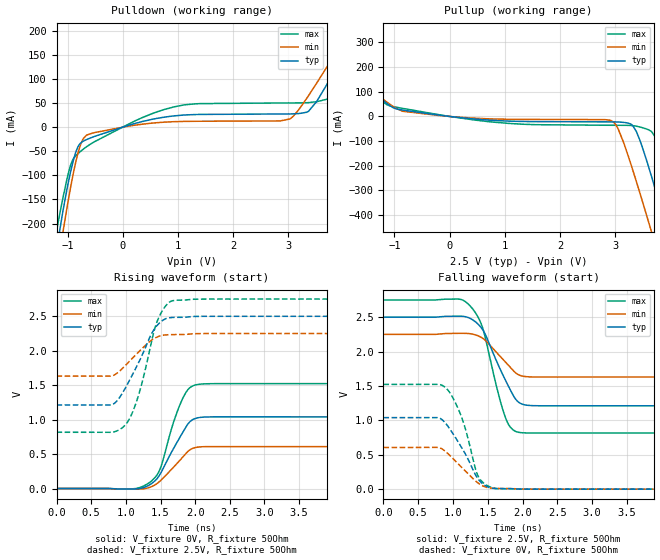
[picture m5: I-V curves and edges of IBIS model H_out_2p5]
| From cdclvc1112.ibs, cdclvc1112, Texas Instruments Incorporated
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|   H_out_2p5
[Model]   H_out_2p5
|Signals :   Y0, Y1, Y2, Y3, Y4, Y5, Y6, Y7, Y8 and Y9
Model_type   Output
Polarity   Non-Inverting
Enable   Active-Low
Vmeas   = 1.21
Vref   = 1.25
Cref   = 2pF
Rref   = 50
|   typ   min   max
C_comp   283fF   269fF   303fF
|C_comp (High state)   176fF   174fF   179fF
[Voltage Range]   2.5   2.25   2.75
[Temperature Range]   25   85   -40
[Pullup Reference]   2.5   2.25   2.75
[Pulldown Reference]   0   0   0
[Power Clamp Reference]   2.5   2.25   2.75
[GND Clamp Reference]   0   0   0
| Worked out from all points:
|   slope of the pulldown table from 0 to 0.375 V, typ, clamps not added: 30.7 ohm
|   slope of the pullup table from 0 to 0.375 V, typ, clamps not added: 43.2 ohm
|   falling waveform, V_fixture 2.5V, R_fixture 50Ohm: 20-80 % time 342ps typ, 337ps min, 282ps max; typ from 2.5 V to 1.21 V
|   rising waveform, V_fixture 0V, R_fixture 50Ohm: 20-80 % time 336ps typ, 340ps min, 279ps max; typ from 0 V to 1.04 V
|   rising waveform, V_fixture 2.5V, R_fixture 50Ohm: 20-80 % time 369ps typ, 373ps min, 297ps max; typ from 1.21 V to 2.5 V
|   falling waveform, V_fixture 0V, R_fixture 50Ohm: 20-80 % time 341ps typ, 361ps min, 268ps max; typ from 1.04 V to 0 V
[Pulldown]
|   Voltage   I(typ)   I(min)   I(max)
-2.5V     -1.296A    -1.308A    -1.284A
-1.206V   -260.7mA   -305.4mA   -220mA
-1.083V   -173.1mA   -216.7mA   -146mA
-853.8mV  -52.8mA    -73.62mA   -59.56mA
-655mV    -25.65mA   -16.52mA   -40.48mA
935mV     23.4mA     11.34mA    42.16mA
3.031V    27.38mA    16.98mA    50.17mA
3.369V    32.99mA    65.5mA     50.86mA
3.71V     90.55mA    126.6mA    58.62mA
4.149V    181.8mA    208.1mA    149.2mA
4.468V    250.2mA    268.2mA    226.3mA
5V        366.5mA    369.8mA    359.1mA
[Pullup]
|   Voltage   I(typ)   I(min)   I(max)
-2.5V     335.9mA    308.3mA    362.8mA
-1.094V   45.6mA     51.2mA     43.52mA
-846.2mV  25.65mA    20.9mA     32.57mA
42.5mV    -1.118mA   -792.6uA   -1.507mA
2.919V    -22.05mA   -15.77mA   -35.77mA
3.065V    -22.61mA   -55.91mA   -35.87mA
3.324V    -38.7mA    -220.3mA   -37.41mA
3.601V    -200.6mA   -424.3mA   -53.6mA
3.732V    -298.6mA   -523.9mA   -87.55mA
3.954V    -470.4mA   -694.2mA   -239.8mA
4.242V    -700.7mA   -919.5mA   -471.5mA
5V        -1.319A    -1.52A     -1.108A
[Ramp]
R_load = 50
|   typ   min   max
dV/dt_r   0.623775/3.36203e-010  0.363855/3.39637e-010  0.913559/2.7929e-010
dV/dt_f   0.772486/3.42455e-010  0.371071/3.371e-010   1.16011/2.82136e-010
[Falling Waveform]
V_fixture = 2.5V
V_fixture_min = 2.25V
V_fixture_max = 2.75V
R_fixture = 50Ohm
C_fixture = 0F
|   Time   V(typ)   V(min)   V(max)
0s        2.5V       2.25V      2.75V
1.072ns   2.514V     2.265V     2.763V
1.23ns    2.49V      2.261V     2.68V
1.425ns   2.32V      2.194V     2.347V
1.643ns   1.824V     1.969V     1.425V
1.755ns   1.581V     1.846V     1.037V
1.823ns   1.445V     1.772V     904.4mV
1.92ns    1.285V     1.676V     832.1mV
2.243ns   1.212V     1.63V      816.4mV
6.248ns   1.213V     1.632V     816.5mV
[Rising Waveform]
V_fixture = 0V
V_fixture_min = 0V
V_fixture_max = 0V
R_fixture = 50Ohm
C_fixture = 0F
|   Time   V(typ)   V(min)   V(max)
0s        3.877nV    3.665nV    2.043nV
1.103ns   -7.291mV   -9.573mV   -3.896mV
1.35ns    57.44mV    18.83mV    93.48mV
1.432ns   123.9mV    60.05mV    174.1mV
1.5ns     217.5mV    114.5mV    299.2mV
1.68ns    565.9mV    300.6mV    936.4mV
1.815ns   804.7mV    449.3mV    1.296V
1.905ns   948.5mV    546.4mV    1.445V
2.01ns    1.019V     595.8mV    1.505V
6.248ns   1.04V      606.4mV    1.523V
[Rising Waveform]
V_fixture = 2.5V
V_fixture_min = 2.25V
V_fixture_max = 2.75V
R_fixture = 50Ohm
C_fixture = 0F
|   Time   V(typ)   V(min)   V(max)
0s        1.213V     1.632V     816.5mV
795ps     1.216V     1.634V     816.3mV
990ps     1.453V     1.783V     920.5mV
1.08ns    1.623V     1.876V     1.069V
1.177ns   1.815V     1.975V     1.336V
1.357ns   2.221V     2.144V     2.072V
1.448ns   2.362V     2.197V     2.414V
1.552ns   2.454V     2.227V     2.621V
1.665ns   2.482V     2.234V     2.723V
6.248ns   2.5V       2.25V      2.75V
[Falling Waveform]
|Gnd
V_fixture = 0V
V_fixture_min = 0V
V_fixture_max = 0V
R_fixture = 50Ohm
C_fixture = 0F
|   Time   V(typ)   V(min)   V(max)
0s        1.04V      606.4mV    1.523V
772.5ps   1.04V      606.5mV    1.524V
900ps     949.7mV    541.5mV    1.468V
1.012ns   786mV      431.6mV    1.301V
1.125ns   603.1mV    316.5mV    1.042V
1.32ns    215.1mV    122.4mV    305.6mV
1.357ns   152.9mV    91.38mV    199.3mV
1.448ns   62.24mV    38.73mV    82.87mV
1.583ns   12.29mV    12.39mV    15.95mV
6.248ns   3.877nV    3.665nV    2.043nV
